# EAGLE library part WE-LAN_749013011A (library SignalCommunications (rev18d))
UtLAN 10/100 Base-T SMD Transformer 1 Port WE-LAN - SMD -- Ethernet -- Power over Ethernet -- 1 Gigabit Ethernet -- Compliant with most IC's for ethernet applications like Intel, AMD, Globespan and Realtek -- Hub, Router, Switch Details see: http://katalog.we-online.de/en/pbs/WE-LAN/S/749010011A? 2016 (C) Würth Elektronik
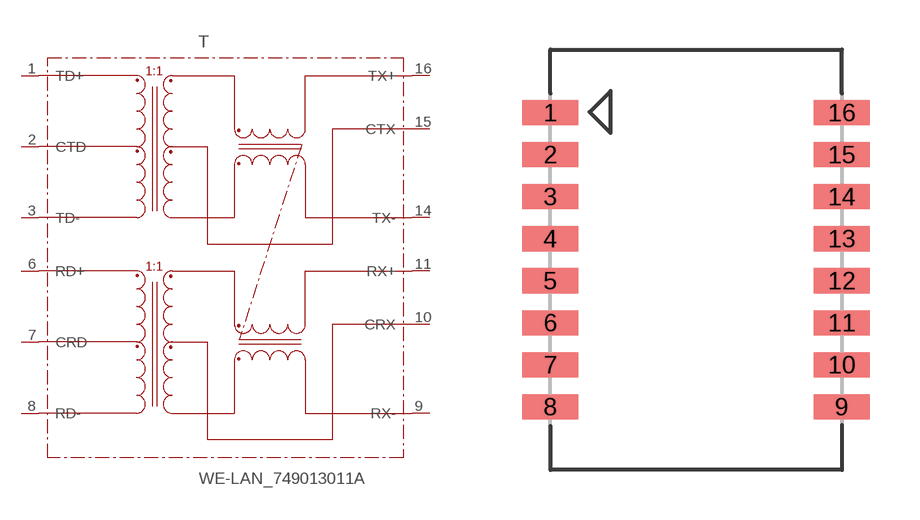
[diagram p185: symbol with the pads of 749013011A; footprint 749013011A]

Designator prefix T

## WE-LAN_749013011A  [749013011A]
1  TD+
2  CTD
3  TD-
6  RD+
7  CRD
8  RD-
9  RX-
10  CRX
11  RX+
14  TX-
15  CTX
16  TX+

## Footprint 749013011A (pad centres in mm)
smd 1.7 x 0.76: 1 -4.4,4.445; 2 -4.4,3.175; 3 -4.4,1.905; 4 -4.4,0.635; 5 -4.4,-0.635; 6 -4.4,-1.905; 7 -4.4,-3.175; 8 -4.4,-4.445; 9 4.4,-4.445; 10 4.4,-3.175; 11 4.4,-1.905; 12 4.4,-0.635; 13 4.4,0.635; 14 4.4,1.905; 15 4.4,3.175; 16 4.4,4.445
